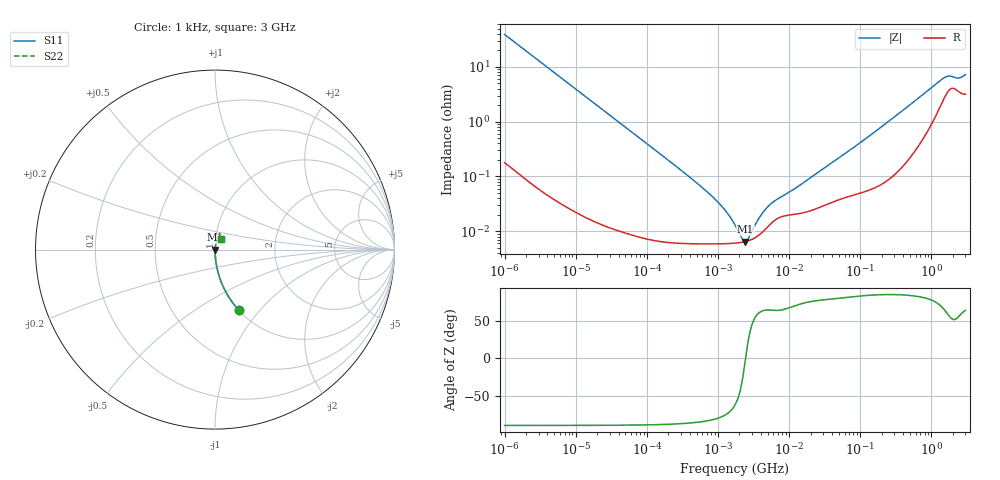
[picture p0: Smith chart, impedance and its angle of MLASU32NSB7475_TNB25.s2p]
! MLASU32NSB7475_TNB25  S-PARAMETER MODEL  ( Standard Model )
! Model Generated by TAIYO YUDEN Corporation (http://www.ty-top.com)
! Version 1.0
! TAIYO YUDEN Control No. 220601
! Copyright(c) 2011 TAIYO YUDEN CO.,LTD. All Rights Reserved.
! Product Description (link to TY-COMPAS)
! https://ds.yuden.co.jp/TYCOMPAS/or/detail?pn=MLASU32NSB7475KTNB25&u=M
! Products Name : Multilayer Ceramic Capacitors
! Characteristics :
!  Capacitance : 4.7 [uF] , Rated Voltage : 50 [V] , TCC : X7R
!  Case Size : 3.2 x 2.5 / 0.126 x 0.098 [mm/inch] , Thickness : 1.9 / 0.075 [mm/inch]
!  (Conditions: Temperature = 25 [degC] , DC Bias Voltage = 0 [V])
! External Node Assignments :
!  1  o---| |---o  2
! GND o---------o GND
! Frequency Range : 1kHz  -  3GHz  [ 401 STEP ]
# MHZ S RI R 50
! Freq[MHz].  S11 Real  S11 Imag  S21 Real  S21 Imag  S12 Real  S12 Imag  S22 Real  S22 Imag
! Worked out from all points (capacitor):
!   401 points, 1 kHz to 3 GHz, reference 50 ohm
!   read as one part in series: C = 4.05 uF near 1.077 kHz
!   lowest |Z| = 6.47 mohm at 2.423 MHz (marker M1)
!   series resonance near 2.439 MHz, so ESL is about 1.1 nH
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0.001  0.1345 -0.339  0.8655 0.339  0.8655 0.339  0.1345 -0.339
0.001685  0.0525 -0.2207  0.9475 0.2207  0.9475 0.2207  0.0525 -0.2207
0.00306  0.0168 -0.1264  0.9832 0.1264  0.9832 0.1264  0.0168 -0.1264
0.01216  0.00125 -0.0324  0.9988 0.0324  0.9988 0.0324  0.00125 -0.0324
0.147855  7.24e-05 -0.00268  0.9999 0.00268  0.9999 0.00268  7.24e-05 -0.00268
0.43594  5.97e-05 -0.000885  0.9999 0.000885  0.9999 0.000885  5.97e-05 -0.000885
0.821683  5.87e-05 -0.000431  0.9999 0.000431  0.9999 0.000431  5.87e-05 -0.000431
1.285341  5.92e-05 -0.000226  0.9999 0.000226  0.9999 0.000226  5.92e-05 -0.000226
1.732051  6.05e-05 -0.000116  0.9999 0.000116  0.9999 0.000116  6.05e-05 -0.000116
2.010629  6.18e-05 -6.46e-05  0.9999 6.46e-05  0.9999 6.46e-05  6.18e-05 -6.46e-05
2.422679  6.46e-05 -2.24e-06  0.9999 2.24e-06  0.9999 2.24e-06  6.46e-05 -2.24e-06
2.812335  6.85e-05 4.8e-05  0.9999 -4.8e-05  0.9999 -4.8e-05  6.85e-05 4.8e-05
3.03007  7.13e-05 7.36e-05  0.9999 -7.36e-05  0.9999 -7.36e-05  7.13e-05 7.36e-05
4.238263  9.69e-05 0.000194  0.9999 -0.000194  0.9999 -0.000194  9.69e-05 0.000194
5.711239  0.000143 0.000295  0.9999 -0.000295  0.9999 -0.000295  0.000143 0.000295
21.06097  0.000243 0.000968  0.9998 -0.000968  0.9998 -0.000968  0.000243 0.000968
83.67817  0.000475 0.00347  0.9995 -0.00347  0.9995 -0.00347  0.000475 0.00347
256.0921  0.001 0.0103  0.999 -0.0103  0.999 -0.0103  0.001 0.0103
1423.198  0.0253 0.0535  0.9747 -0.0535  0.9747 -0.0535  0.0253 0.0535
1780.008  0.0394 0.0525  0.9606 -0.0525  0.9606 -0.0525  0.0394 0.0525
2398.636  0.0368 0.048  0.9632 -0.048  0.9632 -0.048  0.0368 0.048
3000  0.0347 0.0609  0.9653 -0.0609  0.9653 -0.0609  0.0347 0.0609
